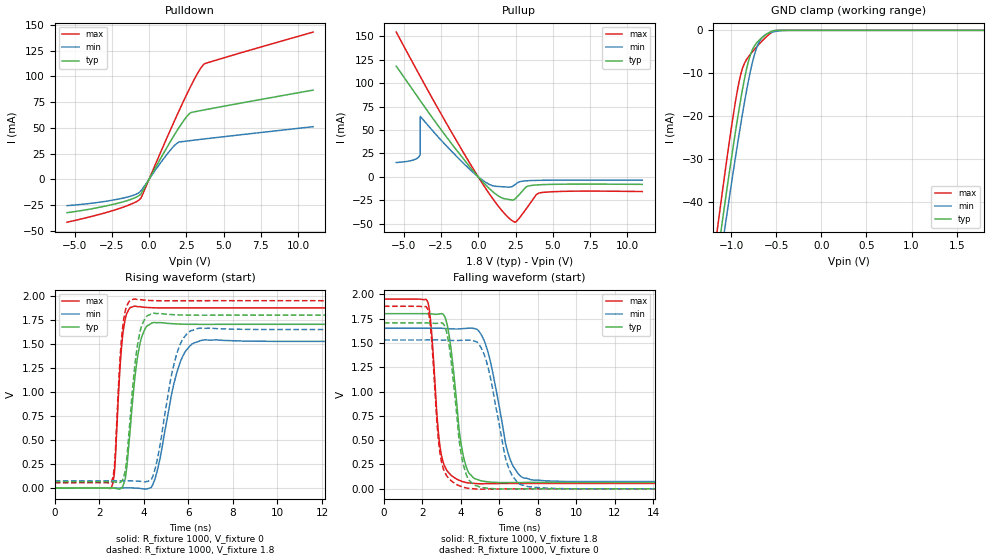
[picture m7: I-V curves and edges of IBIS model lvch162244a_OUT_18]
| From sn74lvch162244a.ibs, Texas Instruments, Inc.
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[Model]   lvch162244a_OUT_18
Model_type  3-state
Enable   Active-Low
Vref =   0
Rref =   1000
Cref =   30p
Vmeas =   0.9
| variable   typ   min   max
C_comp   5.19pF   4.58pF   5.98pF
| C_pullup   3.33pF   2.19pF   6.18pF
| C_pulldown   4.63pF   2.97pF   6.61pF
| C_tri-state   5.19pF   4.58pF   5.98pF
[Temperature Range]   40   100   -40
| Ambient temperature   25   85   -40
[Voltage range]   1.8   1.65   1.95
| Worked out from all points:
|   slope of the pulldown table from 0 to 0.27 V, typ, clamps not added: 37.9 ohm
|   slope of the pullup table from 0 to 0.27 V, typ, clamps not added: 56.7 ohm
|   GND clamp passes 1 mA (typ) near -0.61 V on its own axis
|   rising waveform, R_fixture 1000, V_fixture 0: 20-80 % time 433ps typ, 784ps min, 277ps max; typ from 0 V to 1.7 V
|   falling waveform, R_fixture 1000, V_fixture 1.8: 20-80 % time 577ps typ, 920ps min, 423ps max; typ from 1.8 V to 0.066 V
|   rising waveform, R_fixture 1000, V_fixture 1.8: 20-80 % time 418ps typ, 723ps min, 271ps max; typ from 0.065 V to 1.8 V
|   falling waveform, R_fixture 1000, V_fixture 0: 20-80 % time 570ps typ, 893ps min, 419ps max; typ from 1.71 V to 0 V
[GND Clamp]
| lvch162244a_OUT_18
|   Voltage   I(typ)   I(min)   I(max)
-5.5V     -768.1mA   -753.5mA   -792mA
-1.15V    -52.28mA   -57.69mA   -45.76mA
-1.1V     -44.75mA   -50.35mA   -37.9mA
-1.08V    -41.77mA   -47.45mA   -34.81mA
-1.06V    -38.82mA   -44.57mA   -31.76mA
-950mV    -23.23mA   -29.19mA   -16.22mA
-885mV    -14.93mA   -20.68mA   -9.567mA
-775mV    -5.016mA   -8.387mA   -5.253mA
-710mV    -2.724mA   -3.642mA   -3.667mA
-635mV    -1.318mA   -1.226mA   -2.004mA
-500mV    -22.43uA   -224.3uA   -24.98uA
1.8V      37.81pA    12.24nA    -1.85nA
[Pulldown]
| lvch162244a_OUT_18
|   Voltage   I(typ)   I(min)   I(max)
-5.5V     -32.49mA   -25.65mA   -41.73mA
-2.085V   -23.27mA   -19.34mA   -28.86mA
-1.06V    -18.69mA   -15.64mA   -23.26mA
-580mV    -14.82mA   -11.74mA   -18.83mA
-500mV    -13.22mA   -10.39mA   -17.03mA
1.045V    27.08mA    21.25mA    35.19mA
1.855V    46.72mA    34.73mA    61.57mA
2.395V    58.35mA    36.86mA    78.44mA
2.755V    64.23mA    37.5mA     89.19mA
3.33V     66.33mA    38.5mA     104.8mA
3.695V    67.35mA    39.13mA    111.9mA
11V       86.59mA    51.05mA    143mA
[Pullup]
| lvch162244a_OUT_18
|   Voltage   I(typ)   I(min)   I(max)
-5.5V     118.2mA    15.37mA    154.6mA
-3.935V   82.44mA    22.56mA    108.5mA
-3.895V   81.53mA    24.79mA    107.3mA
-3.89V    81.42mA    64.64mA    107.2mA
185mV     -3.303mA   -2.315mA   -4.644mA
1.375V    -20.6mA    -10.24mA   -31.82mA
2.315V    -24.75mA   -9.98mA    -47.14mA
2.55V     -22.15mA   -7.218mA   -47.62mA
3.225V    -10.56mA   -4.161mA   -33.9mA
3.885V    -8.629mA   -3.728mA   -19.11mA
4.155V    -8.358mA   -3.641mA   -16.97mA
11V       -7.951mA   -3.506mA   -15.62mA
[Ramp]
| lvch162244a_OUT_18
| variable   typ   min   max
dV/dt_r   1.04/4.58E-10   0.93/8.27E-10   1.14/2.87E-10
dV/dt_f   1.04/6.25E-10   0.95/1.01E-09   1.14/4.35E-10
R_load = 1000
[Rising Waveform]
| lvch162244a_OUT_18
R_fixture =   1000
C_fixture =   0
L_fixture =   0
V_fixture =   0
V_fixture_min = 0
V_fixture_max = 0
|   Time   V(typ)   V(min)   V(max)
0s        544.2pV    2.188nV    18.63nV
2.555ns   801.5uV    -109.2uV   12.55mV
2.69ns    -1.319mV   -84.93uV   196.8mV
3.065ns   26.2mV     1.227mV    1.619V
3.56ns    1.065V     646.2uV    1.892V
4.16ns    1.69V      -6.826mV   1.879V
4.585ns   1.72V      165.3mV    1.875V
5.63ns    1.707V     1.309V     1.875V
6.63ns    1.704V     1.539V     1.875V
40ns      1.704V     1.527V     1.875V
[Falling Waveform]
| lvch162244a_OUT_18
R_fixture =   1000
C_fixture =   0
L_fixture =   0
V_fixture =   1.8
V_fixture_min = 1.65
V_fixture_max = 1.95
|   Time   V(typ)   V(min)   V(max)
0s        1.8V       1.65V      1.95V
2.29ns    1.799V     1.65V      1.913V
2.475ns   1.797V     1.65V      1.609V
2.84ns    1.796V     1.65V      556.7mV
3.16ns    1.769V     1.648V     229.9mV
4.225ns   260.5mV    1.648V     66.56mV
5.2ns     77.59mV    1.526V     52.58mV
6.515ns   64.9mV     325.9mV    55.25mV
7.62ns    65.33mV    93.66mV    55.62mV
40ns      65.51mV    74.4mV     55.53mV
[Rising Waveform]
| lvch162244a_OUT_18
R_fixture =   1000
C_fixture =   0
L_fixture =   0
V_fixture =   1.8
V_fixture_min = 1.65
V_fixture_max = 1.95
|   Time   V(typ)   V(min)   V(max)
0s        65.49mV    74.33mV    55.52mV
2.555ns   66.14mV    74.24mV    68.93mV
2.69ns    63.97mV    74.27mV    262.1mV
3.06ns    93.21mV    75.47mV    1.698V
3.545ns   1.161V     74.67mV    1.966V
4.135ns   1.79V      67.97mV    1.954V
4.545ns   1.817V     236.5mV    1.95V
5.525ns   1.802V     1.43V      1.949V
6.435ns   1.799V     1.662V     1.95V
40ns      1.8V       1.65V      1.95V
[Falling Waveform]
| lvch162244a_OUT_18
R_fixture =   1000
C_fixture =   0
L_fixture =   0
V_fixture =   0
V_fixture_min = 0
V_fixture_max = 0
|   Time   V(typ)   V(min)   V(max)
0s        1.705V     1.529V     1.876V
2.29ns    1.705V     1.53V      1.838V
2.47ns    1.703V     1.53V      1.543V
2.83ns    1.702V     1.53V      501.2mV
3.145ns   1.675V     1.528V     177mV
4.225ns   179.1mV    1.528V     10.89mV
5.16ns    11.93mV    1.403V     -3.247mV
6.425ns   -984.4uV   244.4mV    -340.6uV
7.475ns   -175.6uV   22.28mV    77.94uV
40ns      21.59uV    66.8uV     7.689uV
